FUNCTION_BLOCK MIS_EnableMotor
VAR_INPUT
	eCmd : eCommand;
	bEnable : BOOL ;
	iTimeoutMs : INT := 2000;
	
END_VAR
VAR_IN_OUT
	stMisMotorLocal : stMisMotor;	
END_VAR
VAR_OUTPUT
	diError : DINT;
	eStat: ESTATUS;
END_VAR
VAR
	TonTimeout: Ton;
END_VAR

IF eCmd = eCommand.Reset THEN
	diError := 0;
	eStat := eStatus.Done;
	TonTimeout(IN := FALSE,PT := T#0S);//Reset timer 
	RETURN;
END_IF;


CASE eCmd OF
	eCommand.Run:
		TonTimeout(IN := TRUE,PT := ANY_TO_TIME(iTimeoutMs));
		stMisMotorLocal.bEnableMotor := bEnable;
		IF stMisMotorLocal.bEnableMotor AND stMisMotorLocal.State = eDSP402States.OPERATION_ENABLE THEN
			eStat := eStatus.Done;
		ELSIF NOT stMisMotorLocal.bEnableMotor AND stMisMotorLocal.State = eDSP402States.READY_TO_SWITCH_ON THEN
			eStat := eStatus.Done;
		ELSIF TonTimeout.Q THEN
			diError := -1;
			eStat := eStatus.Error;
		END_IF
	ELSE
		eStat := eStatus.Done;
		diError := 0;
		TonTimeout(IN := FALSE,PT := T#0S);//Reset timer 
END_CASE;

END_FUNCTION_BLOCK
